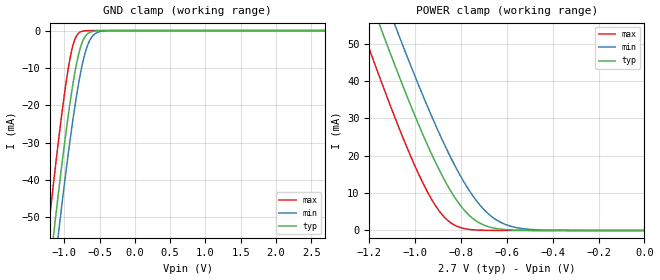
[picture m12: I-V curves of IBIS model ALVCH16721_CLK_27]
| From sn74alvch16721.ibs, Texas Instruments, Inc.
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[Model]   ALVCH16721_CLK_27
Model_type  Input
Vinl=0.8
Vinh=2.0
| variable   typ   min   max
C_comp   1.92pF   1.72pF   2.06pF
[Temperature Range]   40   100   -40
| Ambient temperature   25   85   -40
[Voltage range]   2.7   2.7   2.7
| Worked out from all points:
|   GND clamp passes 1 mA (typ) near -0.68 V on its own axis
|   POWER clamp passes 1 mA (typ) near -0.68 V on its own axis
[GND Clamp]
| ALVCH16721_CLK_27
|   Voltage   I(typ)   I(min)   I(max)
-2.7V     -337.7mA   -347mA     -326.2mA
-1.24V    -69.32mA   -80.17mA   -55.39mA
-1.16V    -55.85mA   -66.73mA   -41.85mA
-1.135V   -51.73mA   -62.6mA    -37.73mA
-1.075V   -42.06mA   -52.87mA   -28.16mA
-985mV    -28.35mA   -38.89mA   -15.11mA
-910mV    -18.08mA   -28.05mA   -6.523mA
-850mV    -11.1mA    -20.16mA   -2.297mA
-775mV    -4.712mA   -11.75mA   -387.5uA
-640mV    -472.1uA   -2.617mA   -10.24uA
-465mV    -14.11uA   -164uA     -86.18nA
2.7V      1.113nA    59.61nA    5.15pA
[POWER Clamp]
| ALVCH16721_CLK_27
|   Voltage   I(typ)   I(min)   I(max)
-2.7V     337.7mA    347mA      326.2mA
-1.23V    67.62mA    78.48mA    53.67mA
-1.15V    54.2mA     65.07mA    40.19mA
-1.08V    42.85mA    53.67mA    28.94mA
-970mV    26.19mA    36.66mA    13.17mA
-880mV    14.42mA    24mA       4.064mA
-835mV    9.584mA    18.33mA    1.666mA
-775mV    4.712mA    11.75mA    387.5uA
-670mV    836.3uA    3.901mA    23.18uA
-595mV    194.7uA    1.357mA    2.999uA
-515mV    38.91uA    377.6uA    337.6nA
-35.59fV  1.113nA    59.61nA    5.15pA
